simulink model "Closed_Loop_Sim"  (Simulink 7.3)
settings: Solver=ode45  StartTime=0.0  StopTime=20  RelTol=1e-3
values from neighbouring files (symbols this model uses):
  Del = diag(ones(1,nunc))    [run.m]
undefined symbols (not defined in the file or in its folder): Au, Bu, Cu, Du, Kl, Kp

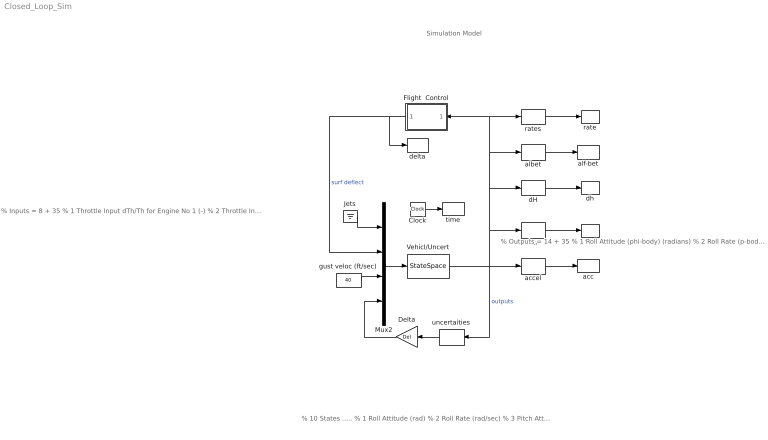
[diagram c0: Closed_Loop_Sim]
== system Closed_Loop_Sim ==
  note: Simulation Model
  note: % 10 States ..... % 1 Roll Attitude (rad) % 2 Roll Rate (rad/sec) % 3 Pitch Attitude (rad) % 4 Pitch Rate (rad/sec) % 5 Yaw Attitude (rad) % 6 Yaw Rate (rad/sec) % 7 Alpha (rad) % 8 Beta (rad) % 9 Delta_Altitude (ft) % 10 Delta_veloc (ft/sec)
  note: % Inputs = 8 + 35 % 1 Throttle Input dTh/Th for Engine No 1 (-) % 2 Throttle Input dTh/Th for Engine No 2 (-) % 3 Throttle Input dTh/Th for Engine No 3 (-) % 4 Elevon Surface No 1 Deflect. (radians) % 5 Aileron Surface No 2 Deflect. (radians) % 6 Rudder-1 Surface No 3 Deflect. (radians) % 7 Rudder-2 Surface No 4 Deflect. (radians) % 8 Wind Gust Azim, Elev Angles=(-135, 90) (deg) % Param Variations = 35 % 9 Cl_beta : 20.000 % Variation % 10 Cm_alfa : 166.667 % Variation % 11 Cn_beta : 30.303 % Variation % 12 Ca_alpha : 22.222 % Variation % 13 Cz_alpha : 10.000 % Variation % 14 Cy_beta : 14.286 % Variation % 15 Cm_0 : -50.000 % Variation % 16 CZ_0 : -2.857 % Variation % 17 Cm_q : -40.000 % Variation % 18 Cz_q : -20.000 % Variation % 19 Cn_p : 54.348 % Variation % 20 Cn_r : -20.408 % Variation % 21 Cl_p : -33.333 % Variation % 22 Cl_r : 25.000 % Variation % 23 CA_0 : -238.095 % Variation % 24 I_xx : 2.857 % Variation % 25 I_yy : 3.333 % Variation % 26 I_zz : 3.030 % Variation % 27 Xcg locat: -1.766 % Variation % 28 Xcg locat: -1.766 % Variation % 29 Ycg locat: 0.5000 Addit. Variat. % 30 Zcg locat: 0.5000 Addit. Variat. % 31 Zcg locat: 0.5000 Addit. Variat. % 32 Ca_surf 1: 18.182 % Variation % 33 Cz_surf 1: 16.667 % Variation % 34 Cm_surf 1: 13.333 % Variation % 35 Cy_surf 2: 500.000 % Variation % 36 Cl_surf 2: 15.000 % Variation % 37 Cn_surf 2: -650.000 % Variation % 38 Cy_surf 3: 10.750 % Variation % 39 Cl_surf 3: 40.000 % Variation % 40 Cn_surf 3: -10.000 % Variation % 41 Cy_surf 4: 5.000 % Variation % 42 Cl_surf 4: 6.250 % Variation % 43 Cn_surf 4: 6.000 % Variation
  note: % Outputs = 14 + 35 % 1 Roll Attitude (phi-body) (radians) % 2 Roll Rate (p-body) (rad/sec) % 3 Pitch Attitude (thet-bdy) (radians) % 4 Pitch Rate (q-body) (rad/sec) % 5 Yaw Attitude (psi-body) (radians) % 6 Yaw Rate (r-body) (rad/sec) % 7 Angle of attack, alfa, (radians) % 8 Angle of sideslip, beta, (radian) % 9 Change in Altitude, delta-h, (feet) % 10 Forward Acceleration (V-dot) (ft/sec) % 11 Cross Range Velocity (Vcr) (ft/sec) % 12 CG Acceleration along X axis, (ft/sec^2) % 13 CG Acceleration along Y axis, (ft/sec^2) % 14 CG Acceleration along Z axis, (ft/sec^2) % Param Variations= 35 % 15 Cl_beta : 20.000 % Variation % 16 Cm_alfa : 166.667 % Variation % 17 Cn_beta : 30.303 % Variation % 18 Ca_alpha : 22.222 % Variation % 19 Cz_alpha : 10.000 % Variation % 20 Cy_beta : 14.286 % Variation % 21 Cm_0 : -50.000 % Variation % 22 CZ_0 : -2.857 % Variation % 23 Cm_q : -40.000 % Variation % 24 Cz_q : -20.000 % Variation % 25 Cn_p : 54.348 % Variation % 26 Cn_r : -20.408 % Variation % 27 Cl_p : -33.333 % Variation % 28 Cl_r : 25.000 % Variation % 29 CA_0 : -238.095 % Variation % 30 I_xx : 2.857 % Variation % 31 I_yy : 3.333 % Variation % 32 I_zz : 3.030 % Variation % 33 Xcg locat: -1.766 % Variation % 34 Xcg locat: -1.766 % Variation % 35 Ycg locat: 0.5000 Addit. Variat. % 36 Zcg locat: 0.5000 Addit. Variat. % 37 Zcg locat: 0.5000 Addit. Variat. % 38 Ca_surf 1: 18.182 % Variation % 39 Cz_surf 1: 16.667 % Variation % 40 Cm_surf 1: 13.333 % Variation % 41 Cy_surf 2: 500.000 % Variation % 42 Cl_surf 2: 15.000 % Variation % 43 Cn_surf 2: -650.000 % Variation % 44 Cy_surf 3: 10.750 % Variation % 45 Cl_surf 3: 40.000 % Variation % 46 Cn_surf 3: -10.000 % Variation % 47 Cy_surf 4: 5.000 % Variation % 48 Cl_surf 4: 6.250 % Variation % 49 Cn_surf 4: 6.000 % Variation
  Clock : Clock
  Delta : Gain  Gain=Del  Multiplication=Matrix(K*u)  ParameterDataType=fixdt(1, 16)  ParameterScaling=2^0  OutDataType=fixdt(1, 16)  OutScaling=2^0
  Flight  Control : Subsystem
  Jets : Ground
  Mux2 : Mux  Inputs=[3, 4, 1, 35]
  Vcr : Selector  InputPortWidth=49  IndexOptions=Index vector (dialog)  Indices=[11]  OutputSizes=1
  Vehicl/Uncert : StateSpace  A=Au  B=Bu  C=Cu  D=Du
  acc : ToWorkspace  VariableName=acc  SampleTime=-1  SaveFormat=Array
  accel : Selector  InputPortWidth=49  IndexOptions=Index vector (dialog)  Indices=[12 13 14]  OutputSizes=1
  albet : Selector  InputPortWidth=49  IndexOptions=Index vector (dialog)  Indices="[7  8]"  OutputSizes=1
  alf-bet : ToWorkspace  VariableName=albet  SampleTime=-1  SaveFormat=Array
  dH : Selector  InputPortWidth=49  IndexOptions=Index vector (dialog)  Indices=[9]  OutputSizes=1
  delta : ToWorkspace  VariableName=delta  SampleTime=-1  SaveFormat=Array
  dh : ToWorkspace  VariableName=dh  SampleTime=-1  SaveFormat=Array
  gust veloc (ft/sec) : Constant  Value=40  OutDataType=sfix(16)  OutScaling=2^0
  rate : ToWorkspace  VariableName=rate  SampleTime=-1  SaveFormat=Array
  rates : Selector  InputPortWidth=49  IndexOptions=Index vector (dialog)  Indices=[2 4 6]  OutputSizes=1
  time : ToWorkspace  VariableName=time  SampleTime=-1  SaveFormat=Array
  uncertaities : Selector  InputPortWidth=49  IndexOptions=Index vector (dialog)  Indices=[15:49]  OutputSizes=1
  vcr : ToWorkspace  VariableName=Vcr  SampleTime=-1  SaveFormat=Array
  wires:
  Jets/1 -> Mux2/1
  gust veloc (ft/sec)/1 -> Mux2/3
  accel/1 -> acc/1
  Vcr/1 -> vcr/1
  dH/1 -> dh/1
  rates/1 -> rate/1
  albet/1 -> alf-bet/1
  Vehicl/Uncert/1 -> accel/1, Vcr/1, dH/1, albet/1, rates/1, Flight  Control/1(in), uncertaities/1  "outputs"
  Delta/1 -> Mux2/4
  Mux2/1 -> Vehicl/Uncert/1
  Flight  Control/1(delta) -> Mux2/2, delta/1  "surf deflect"
  Clock/1 -> time/1
  uncertaities/1 -> Delta/1

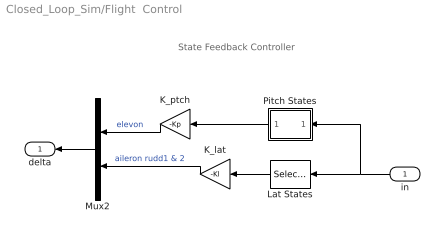
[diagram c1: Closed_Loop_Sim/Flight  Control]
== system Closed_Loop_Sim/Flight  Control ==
  note: State Feedback Controller
  in : Inport
  K_lat : Gain  Gain=-Kl  Multiplication=Matrix(K*u)  ParameterDataType=sfix(16)  ParameterScaling=2^0  OutDataType=sfix(16)  OutScaling=2^0
  K_ptch : Gain  Gain=-Kp  Multiplication=Matrix(K*u)  ParameterDataType=sfix(16)  ParameterScaling=2^0  OutDataType=sfix(16)  OutScaling=2^0
  Lat States : Selector  InputPortWidth=49  IndexOptions=Index vector (dialog)  Indices=[1, 2, 5, 6, 8]  OutputSizes=1
  Mux2 : Mux  Inputs=[1, 3]
  Pitch States : Subsystem
  delta : Outport
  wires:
  Lat States/1 -> K_lat/1
  Pitch States/1(xp) -> K_ptch/1
  K_lat/1 -> Mux2/2  "aileron rudd1 & 2"
  K_ptch/1 -> Mux2/1  "elevon"
  in/1 -> Lat States/1, Pitch States/1(stat)
  Mux2/1 -> delta/1

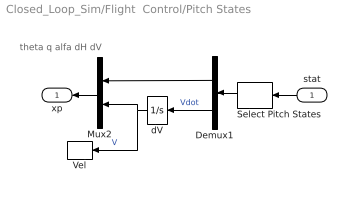
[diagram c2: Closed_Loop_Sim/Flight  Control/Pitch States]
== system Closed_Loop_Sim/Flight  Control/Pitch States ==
  note: theta q alfa dH dV
  stat : Inport  OutDataType=sfix(16)  OutScaling=2^0
  Demux1 : Demux  Outputs=[4,1]
  Mux2 : Mux  Inputs=[4, 1]
  Select Pitch States : Selector  InputPortWidth=49  IndexOptions=Index vector (dialog)  Indices=[3, 4, 7, 9, 10]  OutputSizes=1
  Vel : ToWorkspace  VariableName=dV  SampleTime=-1  SaveFormat=Array
  dV : Integrator
  xp : Outport  OutDataType=sfix(16)  OutScaling=2^0
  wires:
  Select Pitch States/1 -> Demux1/1
  Demux1/2 -> dV/1  "Vdot"
  dV/1 -> Mux2/2, Vel/1  "V"
  Demux1/1 -> Mux2/1
  Mux2/1 -> xp/1
  stat/1 -> Select Pitch States/1
